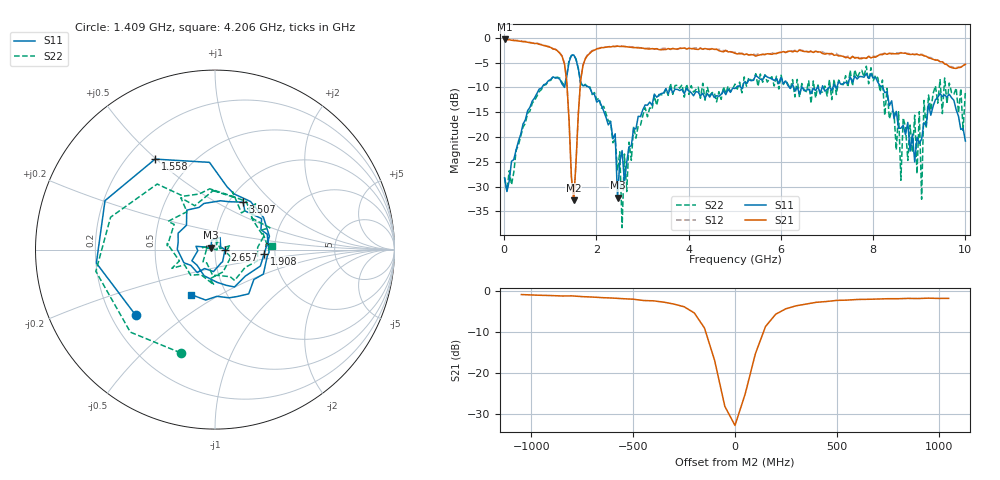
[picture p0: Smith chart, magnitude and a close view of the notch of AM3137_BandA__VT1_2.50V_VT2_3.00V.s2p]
! Date/Time: Tue, Nov 13, 2018 4:48 PM
! Network Analyzer: Agilent Technologies E8364B Rev: A.07.50.67
! Sweep from 0.010 to 10.000 GHz, 201 Points, Sweep Type: LIN
! Power Supply: 2.501 V, -0.001 A
# Hz S DB R 50
!freq MagS11 AngS11 MagS21 AngS21 MagS12 AngS12 MagS22 AngS22
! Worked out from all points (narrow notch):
!   201 points, 10 MHz to 10 GHz, reference 50 ohm
!   highest |S21| = -0.33 dB at 10 MHz (marker M1); lowest = -32.8 dB at 1.508 GHz (marker M2)
!   notch at M2: 29.8 dB deep, 183 MHz wide at half that depth
!   lowest |S11| = -32.2 dB at 2.458 GHz (marker M3), VSWR 1.05, Z = 47.9 + j1.1 ohm
!   |S11| at or under -10 dB: start of sweep to 819.4 MHz; 1.841 GHz to 5.032 GHz (3.191 GHz wide, 92.9 % of centre); 8.207 GHz to end of sweep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
!   |S22| runs from -38.3 to -3.4 dB; largest |S21 - S12| = 0.029
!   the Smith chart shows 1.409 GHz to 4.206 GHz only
!   S11 on the Smith chart (normalised r, x): 1.409 GHz: 0.30, -0.33; 1.558 GHz: 0.31, +0.50; 1.908 GHz: 1.75, -0.08; 2.657 GHz: 1.12, +0.00; 3.507 GHz: 1.16, +0.68; 4.206 GHz: 0.68, -0.37
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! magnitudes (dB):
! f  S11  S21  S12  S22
! 10 MHz  -28.3  -0.3  -0.3  -28.2
! 1.209 GHz  -8.4  -3.1  -3.0  -8.2
! 1.409 GHz  -4.8  -16.9  -16.9  -4.3
! 1.508 GHz  -3.5  -32.8  -32.7  -3.4
! 1.558 GHz  -4.4  -25.1  -25.1  -4.3
! 1.708 GHz  -9.7  -5.6  -5.6  -9.8
! 1.908 GHz  -11.2  -2.7  -2.6  -11.5
! 2.408 GHz  -19.4  -1.8  -1.7  -20.4
! 2.458 GHz  -32.2  -1.7  -1.7  -26.8
! 2.657 GHz  -25.1  -1.8  -1.8  -31.0
! 3.357 GHz  -11.6  -2.4  -2.3  -11.4
! 3.507 GHz  -10.2  -2.4  -2.1  -10.3
! 4.206 GHz  -10.9  -2.4  -2.2  -9.9
! 5.005 GHz  -10.2  -3.1  -2.9  -9.3
! 6.703 GHz  -10.2  -3.0  -2.8  -8.7
! 8.352 GHz  -13.7  -3.1  -3.1  -16.3
! 8.551 GHz  -18.2  -3.2  -3.1  -14.9
! 8.601 GHz  -18.2  -3.0  -3.0  -28.7
! 9.001 GHz  -21.3  -3.5  -3.4  -14.9
! 9.051 GHz  -20.4  -3.4  -3.3  -32.6
! 9.101 GHz  -17.1  -3.6  -3.6  -12.6
! 10 GHz  -20.8  -5.4  -5.2  -10.7
